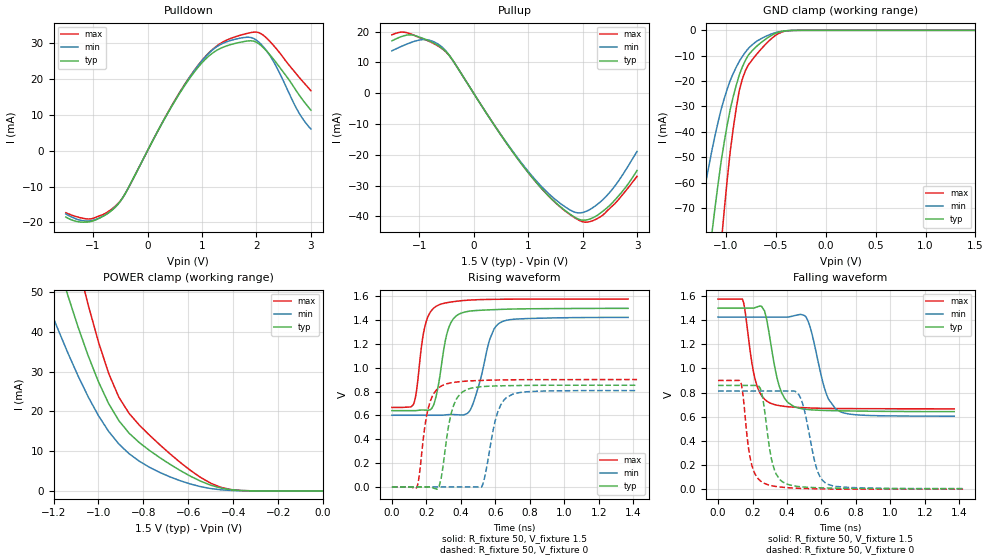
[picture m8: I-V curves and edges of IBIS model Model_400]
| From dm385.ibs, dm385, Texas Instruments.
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| Model based on original model for BCSHTLTCSCDDVPBFZ_SSDHV
|   Sub model SR00_10MA_PADP_5PER_1P5
[model]   Model_400
|[Description]  [1.5V-3-STATE-NOTERM-FASTEST:10MA, IND, 5%]
|   Fastest slew rate (SR[1:0] = "00"), 0.80 * RExt = 1.250 * Iout
|   (I[2:0] = "101"), 10mA nominal with Rext = 50R,ODT off (ODT[1:0]
|   = "00") CMOS mode,Industrial temperature range (-40C to 125C,
|   25C nominal),5% power supply tolerance
|[Input Load]   NOTERM
|[Output Drive] FASTEST:10MA
|Voltage   1.5V
|Mode   3-STATE
Model_type   3-state
Polarity   Non-Inverting
Enable   Active-Low
Cref =  15pF
Rref =  100.0000M
Vref =  0V
Vmeas =  0.75
C_comp   1.865048p   1.679967p   1.989968p
[Temperature Range]   25   125   -40
[Voltage Range]   1.5   1.425   1.575
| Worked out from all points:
|   slope of the pulldown table from 0 to 0.225 V, typ, clamps not added: 34.7 ohm
|   slope of the pullup table from 0 to 0.225 V, typ, clamps not added: 36.1 ohm
|   GND clamp passes 1 mA (typ) near -0.49 V on its own axis
|   POWER clamp passes 1 mA (typ) near -0.47 V on its own axis
|   rising waveform, R_fixture 50, V_fixture 1.5: 20-80 % time 63.7ps typ, 87.2ps min, 54ps max; typ from 0.64 V to 1.5 V
|   rising waveform, R_fixture 50, V_fixture 0: 20-80 % time 61.5ps typ, 70.1ps min, 57.9ps max; typ from 0 V to 0.852 V
|   falling waveform, R_fixture 50, V_fixture 1.5: 20-80 % time 73ps typ, 84.9ps min, 63.6ps max; typ from 1.5 V to 0.643 V
|   falling waveform, R_fixture 50, V_fixture 0: 20-80 % time 57.6ps typ, 71.7ps min, 50.4ps max; typ from 0.86 V to 0.004 V
[POWER_clamp]
-1.5V     126mA      88.76mA    168.8mA
-1.242V   69.8mA     49.43mA    94.36mA
-1.136V   49.16mA    34.7mA     67.53mA
-1.061V   36.35mA    25.39mA    50.04mA
-1.045V   33.92mA    23.62mA    46.67mA
-954.5mV  21.93mA    14.94mA    29.52mA
-909.1mV  17.64mA    11.78mA    23.53mA
-863.6mV  14.51mA    9.346mA    19.48mA
-772.7mV  10.16mA    5.937mA    14mA
-590.9mV  3.705mA    1.741mA    5.168mA
-454.5mV  710.5uA    279.1uA    892.2uA
0V        1.424nA    14.75nA    2.169nA
[Pulldown]
-1.5V     -18.53mA   -17.67mA   -17.32mA
-1.045V   -19.8mA    -19.56mA   -19.06mA
-545.5mV  -15.01mA   -15.01mA   -14.82mA
-409.1mV  -11.96mA   -11.99mA   -12.02mA
727.3mV   19.21mA    19.5mA     19.59mA
1.136V    26.61mA    27.42mA    27.53mA
1.455V    29.32mA    30.47mA    30.93mA
1.864V    30.73mA    31.72mA    32.92mA
2.091V    29.33mA    29.67mA    32.66mA
2.318V    25.5mA     24.82mA    29.36mA
2.773V    15.82mA    10.78mA    20.73mA
3V        11.34mA    6.07mA     16.76mA
[Pullup]
-1.5V     17mA       13.76mA    18.94mA
-1.136V   18.91mA    16.54mA    19.11mA
-863.6mV  17.34mA    17.36mA    17.19mA
-590.9mV  14.75mA    15.13mA    14.58mA
-409.1mV  11.37mA    11.36mA    11.3mA
954.5mV   -24.69mA   -24.32mA   -24.66mA
1.409V    -33.89mA   -33.1mA    -33.96mA
1.818V    -39.82mA   -38.34mA   -39.98mA
2.045V    -41.2mA    -38.48mA   -41.86mA
2.318V    -39.01mA   -35.4mA    -40.21mA
2.636V    -33.81mA   -29.06mA   -34.99mA
3V        -25.08mA   -18.91mA   -26.96mA
[GND_clamp]
-1.5V     -219.3mA   -131.6mA   -364.3mA
-1.288V   -134.4mA   -79.74mA   -225.6mA
-1.258V   -122.9mA   -72.77mA   -206.3mA
-1.136V   -79.27mA   -46.88mA   -132.4mA
-1.045V   -51.5mA    -31.06mA   -84.11mA
-1.015V   -44.02mA   -26.9mA    -70.91mA
-954.5mV  -31.01mA   -19.7mA    -47.55mA
-863.6mV  -17.48mA   -12.16mA   -23.55mA
-803mV    -11.81mA   -8.597mA   -15.85mA
-681.8mV  -5.986mA   -4.096mA   -9.026mA
-378.8mV  -126.2uA   -131.8uA   -179.7uA
1.5V      1.424nA    36.56nA    1.506nA
[Ramp]
dV/dt_f 0.52683538/74.107425p 0.50719508/86.759149p 0.55340338/63.751694p
dV/dt_r 0.52645567/63.068431p 0.50524027/71.351331p 0.54898106/57.866008p
R_load = 50
[Rising Waveform]
R_fixture = 50
V_fixture = 1.5
V_fixture_min = 1.425
V_fixture_max = 1.575
0s        639.5mV    601mV      666.5mV
124.4ps   639.5mV    601mV      690.3mV
194.1ps   644mV      601mV      1.361V
272.7ps   878.6mV    601mV      1.526V
316.6ps   1.271V     604.8mV    1.544V
356.9ps   1.41V      606.9mV    1.553V
457ps     1.475V     652.1mV    1.567V
567.7ps   1.485V     1.239V     1.572V
626.1ps   1.488V     1.376V     1.573V
1.37ns    1.497V     1.421V     1.575V
[Rising Waveform]
R_fixture = 50
V_fixture = 0
V_fixture_min = 0
V_fixture_max = 0
0s        0V         0V         0V
144.1ps   0V         0V         -5.834mV
209.1ps   0V         0V         649.5mV
295.5ps   164.3mV    0V         852.5mV
355.4ps   673.2mV    0V         875.7mV
437.1ps   818.2mV    0V         887.6mV
521ps     840.8mV    0V         893mV
600ps     846.3mV    559.7mV    896.1mV
664.3ps   848.6mV    748.6mV    897.7mV
1.422ns   852.5mV    807.9mV    900.3mV
[Falling Waveform]
R_fixture = 50
V_fixture = 1.5
V_fixture_min = 1.425
V_fixture_max = 1.575
0s        1.501V     1.426V     1.575V
141ps     1.501V     1.426V     1.575V
217.5ps   1.506V     1.426V     896.8mV
269.7ps   1.478V     1.426V     745.2mV
305.8ps   1.207V     1.426V     711.7mV
370.5ps   794.3mV    1.426V     688.8mV
507.6ps   662mV      1.43V      674.4mV
628.8ps   651.7mV    786.7mV    669.2mV
699.8ps   649.5mV    648.4mV    668.1mV
1.37ns    642.7mV    604.8mV    665.7mV
[Falling Waveform]
R_fixture = 50
V_fixture = 0
V_fixture_min = 0
V_fixture_max = 0
0s        859.7mV    813mV      900.8mV
132.2ps   859.7mV    813mV      883.4mV
193.5ps   859.7mV    813mV      212.3mV
271.9ps   632.2mV    813mV      46.23mV
328.5ps   154.8mV    813mV      23.8mV
408.1ps   38.05mV    813mV      11.73mV
477.4ps   20.25mV    759.3mV    6.507mV
573ps     12.24mV    166.1mV    3.321mV
635.6ps   9.779mV    40.8mV     2.273mV
1.422ns   3.74mV     5.177mV    0V
